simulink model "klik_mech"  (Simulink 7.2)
settings: Solver=ode45  StartTime=0.0  StopTime=10.0  MaxStep=0.05  RelTol=1e-3
InitFcn:
  | init_klik;
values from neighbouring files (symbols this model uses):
  L1 = 1.5    [init_klik.m]    (also in init_ctyrkloub.m = 3; init_withworth.m = 2)
  L2 = v/sin(uhel3)    [init_klik.m]    (also in init_ctyrkloub.m = 5; init_withworth.m = 5)
  L3 = L1/(sin(uhel1))    [init_klik.m]    (also in init_ctyrkloub.m = 0.5)
  omega = 5    [init_klik.m]    (also in init_ctyrkloub.m = 1; init_withworth.m = 0.5)
  uhel1 = (pi/180)*fi    (= 1.3962634016)    [init_klik.m]
undefined symbols (not defined in the file or in its folder): deg, kg, m, N, rad, s
libraries: mblibv1 x13, simulink x3

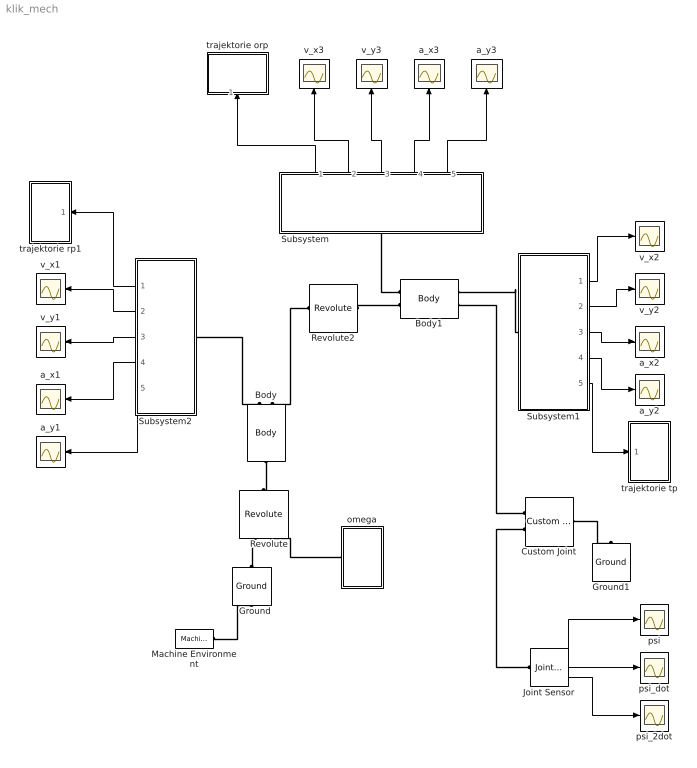
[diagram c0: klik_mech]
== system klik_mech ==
  Body : mblibv1/Bodies/Body  Orientation=up  DialogController=MECH.DynMechDlgSource  PhysicalDomain=mechanical  SubClassName=Unknown  LeftPortType=workingframe  RightPortType=workingframe  LConnTagsString=CS1  RConnTagsString=CS3|CS2  UpdateFromCAD=off  DialogClass=MechanicalBodyBlock  Mass=1  MassUnits=kg  InertiaUnits=kg*m^2  Inertia=eye(3)  Shape=Cylinder  ShapeDims=[1 1]  ShapeUnits=m  ShapeUse=false  Density=1  DensityUnits=kg/m^3  DensityUse=false  GraphicsMode=MACHINE_DEFAULT  BodyColorSelMode=MACHINE_DEFAULT  BodyColor=[1 0 0]  AttachedToCS=CG  CG=Left$CG$[L1/2 0 0]$CS1$CS1$m$[0 0 uhel1]$Euler X-Y-Z$rad$WORLD$false$none  WorkingFrames=Right$CS3$[0 0 0]$CS2$CS2$m$[0 0 uhel1]$Euler X-Y-Z$rad$WORLD$true$none#Left$CS1$[0 0 0]$Adjoining$Adjoining$m$[0 0 uhel1]$Euler X-Y-Z$rad$WORLD$true$none#Right$CS2$[L1 0 0]$CS1$CS1$m$[0 0 uhel1]$Euler X-Y-Z$rad$WORLD$true$none  CGPos=[L1/2 0 0]  CGRot=[0 0 uhel1]  CS0Pos=[]  CS0Rot=[]  CS1Pos=[0 0 0]  CS1Rot=[0 0 uhel1]  CS2Pos=[L1 0 0]  CS2Rot=[0 0 uhel1]  CS3Pos=[0 0 0]  CS3Rot=[0 0 uhel1]  CS4Pos=[]  CS4Rot=[]  CS5Pos=[]  CS5Rot=[]  CS6Pos=[]  CS6Rot=[]  CS7Pos=[]  CS7Rot=[]  CS8Pos=[]  CS8Rot=[]  CS9Pos=[]  CS9Rot=[]  CS10Pos=[]  CS10Rot=[]  CS11Pos=[]  CS11Rot=[]  CS12Pos=[]  CS12Rot=[]  CS13Pos=[]  CS13Rot=[]  CS14Pos=[]  CS14Rot=[]  CS15Pos=[]  CS15Rot=[]  CS16Pos=[]  CS16Rot=[]  CS17Pos=[]  CS17Rot=[]  CS18Pos=[]  CS18Rot=[]  CS19Pos=[]  CS19Rot=[]  CS20Pos=[]  CS20Rot=[]
  Body1 : mblibv1/Bodies/Body  DialogController=MECH.DynMechDlgSource  PhysicalDomain=mechanical  SubClassName=Unknown  LeftPortType=workingframe  RightPortType=workingframe  LConnTagsString=CG|CS1  RConnTagsString=CS3|CS2  UpdateFromCAD=off  DialogClass=MechanicalBodyBlock  Mass=1  MassUnits=kg  InertiaUnits=kg*m^2  Inertia=eye(3)  Shape=Cylinder  ShapeDims=[1 1]  ShapeUnits=m  ShapeUse=false  Density=1  DensityUnits=kg/m^3  DensityUse=false  GraphicsMode=MACHINE_DEFAULT  BodyColorSelMode=MACHINE_DEFAULT  BodyColor=[1 0 0]  AttachedToCS=CG  CG=Left$CG$[L2/2 0 0]$CS1$CS1$m$[0 0 0]$Euler X-Y-Z$rad$CS1$true$none  WorkingFrames=Right$CS3$[0 0 0]$CS2$CS2$m$[0 0 0]$Euler X-Y-Z$rad$CS1$true$none#Left$CS1$[0 0 0]$Adjoining$Adjoining$m$[0 0 3*pi/2]$Euler X-Y-Z$rad$Adjoining$true$none#Right$CS2$[L2 0 0]$CS1$CS1$m$[0 0 0]$Euler X-Y-Z$rad$CS1$true$none  CGPos=[L2/2 0 0]  CGRot=[0 0 0]  CS0Pos=[]  CS0Rot=[]  CS1Pos=[0 0 0]  CS1Rot=[0 0 3*pi/2]  CS2Pos=[L2 0 0]  CS2Rot=[0 0 0]  CS3Pos=[0 0 0]  CS3Rot=[0 0 0]  CS4Pos=[]  CS4Rot=[]  CS5Pos=[]  CS5Rot=[]  CS6Pos=[]  CS6Rot=[]  CS7Pos=[]  CS7Rot=[]  CS8Pos=[]  CS8Rot=[]  CS9Pos=[]  CS9Rot=[]  CS10Pos=[]  CS10Rot=[]  CS11Pos=[]  CS11Rot=[]  CS12Pos=[]  CS12Rot=[]  CS13Pos=[]  CS13Rot=[]  CS14Pos=[]  CS14Rot=[]  CS15Pos=[]  CS15Rot=[]  CS16Pos=[]  CS16Rot=[]  CS17Pos=[]  CS17Rot=[]  CS18Pos=[]  CS18Rot=[]  CS19Pos=[]  CS19Rot=[]  CS20Pos=[]  CS20Rot=[]
  Custom Joint : mblibv1/Joints/Custom Joint  DialogController=MECH.DynMechDlgSource  PhysicalDomain=mechanical  SubClassName=custom_joint  LeftPortType=blob  RightPortType=blob  LConnTagsString=__newl0|SA1  RConnTagsString=__newr0  UpdateFromCAD=off  NumSAPorts=1  CutJoint=off  MarkAsCut=off  Primitives=prismatic  PrimitiveProps=R1$World$[0 0 1]$Revolute#P1$World$[1 0 0]$Prismatic  DialogClass=JointBlock  R1Axis=[0 0 1]  R2Axis=[]  R3Axis=[]  P1Axis=[1 0 0]  P2Axis=[]  P3Axis=[]  SAxis=[]
  Ground : mblibv1/Bodies/Ground  Orientation=up  DialogController=MECH.DynMechDlgSource  SystemSampleTime=-1  UpdateFromCAD=off  LeftPortType=env  RightPortType=workingframe  PhysicalDomain=Mechanical  DialogClass=GroundBlock  CoordPosition=[0 0 0]  CoordPositionUnits=m  StateVectorMgrId=4  MachineId=[5 0]  ShowEnvPort=on
  Ground1 : mblibv1/Bodies/Ground  Orientation=up  DialogController=MECH.DynMechDlgSource  SystemSampleTime=-1  UpdateFromCAD=off  LeftPortType=env  RightPortType=workingframe  PhysicalDomain=Mechanical  DialogClass=GroundBlock  CoordPosition=[L3 0 0]  CoordPositionUnits=m  StateVectorMgrId=-1  MachineId=[0 0]  ShowEnvPort=off
  Joint Sensor : mblibv1/Sensors &  Actuators/Joint Sensor  DialogController=MECH.DynMechDlgSource  SystemSampleTime=-1  UpdateFromCAD=off  PhysicalDomain=Mechanical  PortType=blob  Muxed=off  Pose=off  Angle=on  AngleUnits=rad  ArcVelocity=on  ArcVelocityUnits=rad/s  ArcAcceleration=on  ArcAccelerationUnits=rad/s^2  CoordPosition=on  CoordPositionUnits=m  Velocity=off  VelocityUnits=m/s  Acceleration=off  AccelerationUnits=m/s^2  Quaternion=on  QuaternionDT=off  QuaternionDDT=off  QuaternionUnits=off  OutputVector=[1]  ActiveIO=on  Width=3  DialogClass=MechanicalSensorBlock  Primitive=R1  Force=off  ForceUnits=N  Torque=off  TorqueUnits=N*m  ReferenceFrame=Absolute (World)  ReactionSensedSide=Base  ReactionReferenceFrame=Absolute (World)  ReactionForce=off  ReactionForceUnits=N  ReactionMoment=off  ReactionMomentUnits=N*m
  Machine Environment : mblibv1/Bodies/Machine Environment  DialogController=MECH.DialogSource  SystemSampleTime=-1  PortType=env  PhysicalDomain=Mechanical  DialogTemplateClass=MECH.MachineEnvironment  SyncWhenCopied=off  Gravity=[0 -9.81 0]  GravityUnits=m/s^2  GravityAsSignal=off  Dimensionality=Auto-detect  AnalysisType=Kinematics  LinearAssemblyTolerance=1e-3  LinearAssemblyToleranceUnits=m  AngularAssemblyTolerance=1e-3  AngularAssemblyToleranceUnits=rad  ConstraintSolverType=Stabilizing  ConstraintRelTolerance=1e-4  ConstraintAbsTolerance=1e-4  UseRobustSingularityHandling=off  RedundancyAnalysisToleranceType=Automatically select tolerance  RedundancyAnalysisTolerance=1e-14  StatePerturbationType=Fixed  PerturbationSize=1e-5  VisualizeMachine=on  BodyVisualizationType=Use model default body geometries  BodyColorSelMode=Use model default  DefaultBodyColor=[1 0 0]
  Revolute : mblibv1/Joints/Revolute  Orientation=up  DialogController=MECH.DynMechDlgSource  PhysicalDomain=mechanical  SubClassName=Unknown  LeftPortType=blob  RightPortType=blob  LConnTagsString=__newl0|SA1  RConnTagsString=__newr0  UpdateFromCAD=off  NumSAPorts=1  CutJoint=off  MarkAsCut=off  Primitives=prismatic  PrimitiveProps=R1$World$[0 0 1]$revolute  DialogClass=JointBlock  R1Axis=[0 0 1]
  Revolute2 : mblibv1/Joints/Revolute  DialogController=MECH.DynMechDlgSource  PhysicalDomain=mechanical  SubClassName=Unknown  LeftPortType=blob  RightPortType=blob  LConnTagsString=__newl0  RConnTagsString=__newr0  UpdateFromCAD=off  NumSAPorts=0  CutJoint=off  MarkAsCut=off  Primitives=prismatic  PrimitiveProps=R1$WORLD$[0 0 1]$revolute  DialogClass=JointBlock  R1Axis=[0 0 1]
  Subsystem : Subsystem  Orientation=up
  Subsystem1 : Subsystem
  Subsystem2 : Subsystem  Orientation=left
  a_x1 : Scope
  a_x2 : Scope
  a_x3 : Scope
  a_y1 : Scope
  a_y2 : Scope
  a_y3 : Scope
  omega : Subsystem  Orientation=left
  psi : Scope
  psi_2dot : Scope
  psi_dot : Scope
  trajektorie orp : Subsystem  Orientation=up
  trajektorie rp1 : Subsystem  Orientation=left
  trajektorie tp : Subsystem
  v_x1 : Scope
  v_x2 : Scope
  v_x3 : Scope
  v_y1 : Scope
  v_y2 : Scope
  v_y3 : Scope
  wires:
  Joint Sensor/1 -> psi/1
  Subsystem1/1(Out1) -> v_x2/1
  Subsystem1/2(Out2) -> v_y2/1
  Subsystem1/3(Out3) -> a_x2/1
  Subsystem1/4(Out4) -> a_y2/1
  Subsystem1/5(Out5) -> trajektorie tp/1(In1)
  Subsystem/1(Out1) -> trajektorie orp/1(In1)
  Subsystem/2(Out2) -> v_x3/1
  Subsystem/3(Out3) -> v_y3/1
  Subsystem/4(Out4) -> a_x3/1
  Subsystem/5(Out5) -> a_y3/1
  Subsystem2/1(Out1) -> trajektorie rp1/1(In1)
  Subsystem2/2(Out2) -> v_x1/1
  Subsystem2/3(Out3) -> v_y1/1
  Subsystem2/4(Out4) -> a_x1/1
  Subsystem2/5(Out5) -> a_y1/1
  Joint Sensor/2 -> psi_dot/1
  Joint Sensor/3 -> psi_2dot/1
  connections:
  Subsystem2/LConn1 -- Body/RConn1
  Ground/RConn1 -- Revolute/LConn1
  omega/RConn1 -- Revolute/LConn2
  Subsystem/LConn1 -- Body1/LConn1
  Custom Joint/LConn1 -- Body1/RConn2
  Revolute2/LConn1 -- Body/RConn2
  Subsystem1/LConn1 -- Body1/RConn1
  Body/LConn1 -- Revolute/RConn1
  Revolute2/RConn1 -- Body1/LConn2
  Joint Sensor/LConn1 -- Custom Joint/LConn2
  Machine Environment/RConn1 -- Ground/LConn1
  Custom Joint/RConn1 -- Ground1/RConn1

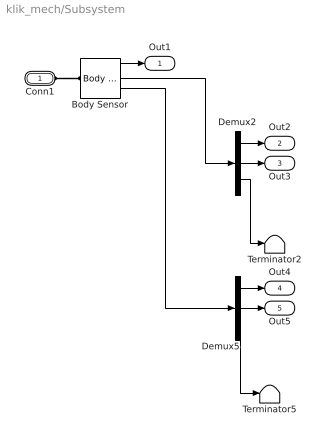
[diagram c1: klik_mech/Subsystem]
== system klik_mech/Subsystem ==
  Body Sensor : mblibv1/Sensors &  Actuators/Body Sensor  DialogController=MECH.DynMechDlgSource  SystemSampleTime=-1  UpdateFromCAD=off  PhysicalDomain=Mechanical  PortType=blob  Muxed=off  Pose=off  Angle=on  AngleUnits=deg  ArcVelocity=off  ArcVelocityUnits=deg/s  ArcAcceleration=off  ArcAccelerationUnits=deg/s^2  CoordPosition=on  CoordPositionUnits=m  Velocity=on  VelocityUnits=m/s  Acceleration=on  AccelerationUnits=m/s^2  Quaternion=on  QuaternionDT=off  QuaternionDDT=off  QuaternionUnits=off  OutputVector=[1]  ActiveIO=on  Width=9  DialogClass=MechanicalSensorBlock  ReferenceFrame=Absolute (World)
  Demux2 : Demux  Outputs=3
  Demux5 : Demux  Outputs=3
  Terminator2 : Terminator
  Terminator5 : Terminator
  Conn1 : PMIOPort  Port=1  Side=Left
  Out1 : Outport
  Out2 : Outport  Port=2
  Out3 : Outport  Port=3
  Out4 : Outport  Port=4
  Out5 : Outport  Port=5
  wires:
  Body Sensor/2 -> Demux2/1
  Demux2/3 -> Terminator2/1
  Demux5/3 -> Terminator5/1
  Body Sensor/3 -> Demux5/1
  Body Sensor/1 -> Out1/1
  Demux2/1 -> Out2/1
  Demux2/2 -> Out3/1
  Demux5/1 -> Out4/1
  Demux5/2 -> Out5/1
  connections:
  Conn1/RConn1 -- Body Sensor/LConn1

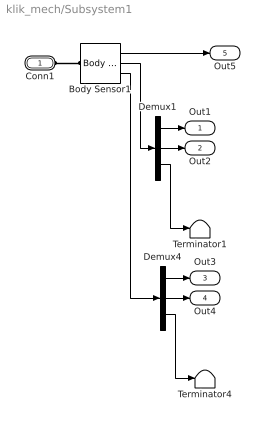
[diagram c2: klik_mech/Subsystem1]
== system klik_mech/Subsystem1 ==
  Body Sensor1 : mblibv1/Sensors &  Actuators/Body Sensor  DialogController=MECH.DynMechDlgSource  SystemSampleTime=-1  UpdateFromCAD=off  PhysicalDomain=Mechanical  PortType=blob  Muxed=off  Pose=off  Angle=on  AngleUnits=deg  ArcVelocity=off  ArcVelocityUnits=deg/s  ArcAcceleration=off  ArcAccelerationUnits=deg/s^2  CoordPosition=on  CoordPositionUnits=m  Velocity=on  VelocityUnits=m/s  Acceleration=on  AccelerationUnits=m/s^2  Quaternion=on  QuaternionDT=off  QuaternionDDT=off  QuaternionUnits=off  OutputVector=[1]  ActiveIO=on  Width=9  DialogClass=MechanicalSensorBlock  ReferenceFrame=Absolute (World)
  Demux1 : Demux  Outputs=3
  Demux4 : Demux  Outputs=3
  Terminator1 : Terminator
  Terminator4 : Terminator
  Conn1 : PMIOPort  Port=1  Side=Left
  Out1 : Outport
  Out2 : Outport  Port=2
  Out3 : Outport  Port=3
  Out4 : Outport  Port=4
  Out5 : Outport  Port=5
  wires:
  Body Sensor1/1 -> Out5/1
  Demux1/3 -> Terminator1/1
  Body Sensor1/2 -> Demux1/1
  Demux4/3 -> Terminator4/1
  Body Sensor1/3 -> Demux4/1
  Demux1/1 -> Out1/1
  Demux1/2 -> Out2/1
  Demux4/1 -> Out3/1
  Demux4/2 -> Out4/1
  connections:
  Conn1/RConn1 -- Body Sensor1/LConn1

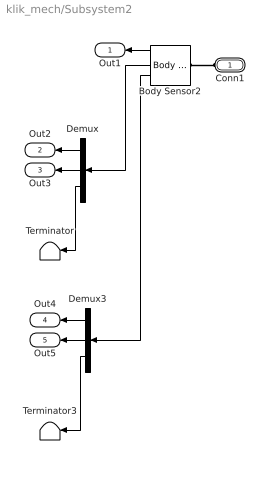
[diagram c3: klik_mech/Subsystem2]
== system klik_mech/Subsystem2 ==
  Body Sensor2 : mblibv1/Sensors &  Actuators/Body Sensor  Orientation=left  DialogController=MECH.DynMechDlgSource  SystemSampleTime=-1  UpdateFromCAD=off  PhysicalDomain=Mechanical  PortType=blob  Muxed=off  Pose=off  Angle=on  AngleUnits=deg  ArcVelocity=off  ArcVelocityUnits=deg/s  ArcAcceleration=off  ArcAccelerationUnits=deg/s^2  CoordPosition=on  CoordPositionUnits=m  Velocity=on  VelocityUnits=m/s  Acceleration=on  AccelerationUnits=m/s^2  Quaternion=on  QuaternionDT=off  QuaternionDDT=off  QuaternionUnits=off  OutputVector=[1]  ActiveIO=on  Width=9  DialogClass=MechanicalSensorBlock  ReferenceFrame=Absolute (World)
  Demux : Demux  Orientation=left  Outputs=3
  Demux3 : Demux  Orientation=left  Outputs=3
  Terminator : Terminator
  Terminator3 : Terminator
  Conn1 : PMIOPort  Orientation=left  Port=1  Side=Left
  Out1 : Outport  Orientation=left
  Out2 : Outport  Orientation=left  Port=2
  Out3 : Outport  Orientation=left  Port=3
  Out4 : Outport  Orientation=left  Port=4
  Out5 : Outport  Orientation=left  Port=5
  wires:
  Demux/3 -> Terminator/1
  Body Sensor2/2 -> Demux/1
  Demux3/3 -> Terminator3/1
  Body Sensor2/3 -> Demux3/1
  Body Sensor2/1 -> Out1/1
  Demux/1 -> Out2/1
  Demux/2 -> Out3/1
  Demux3/1 -> Out4/1
  Demux3/2 -> Out5/1
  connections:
  Conn1/RConn1 -- Body Sensor2/LConn1

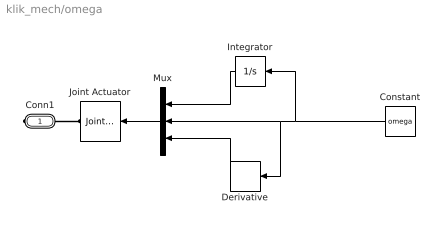
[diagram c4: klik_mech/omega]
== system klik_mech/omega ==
  Constant : Constant  Orientation=left  Value=omega  OutDataType=sfix(16)  OutScaling=2^0
  Derivative : Derivative  Orientation=left
  Integrator : Integrator  Orientation=left
  Joint Actuator : mblibv1/Sensors &  Actuators/Joint Actuator  Orientation=left  DialogController=MECH.DynMechDlgSource  SystemSampleTime=-1  UpdateFromCAD=off  PhysicalDomain=Mechanical  PortType=blob  ActuationStyle=Motion  AngleUnits=rad  ArcVelocityUnits=rad/s  ArcAccelerationUnits=rad/s^2  CoordPositionUnits=m  VelocityUnits=m/s  AccelerationUnits=m/s^2  ForceUnits=N  TorqueUnits=N*m  ActiveIO=on  Width=3  DialogClass=MechanicalActuatorBlock  Primitive=R1  ReferenceFrame=Absolute (World)
  Mux : Mux  Orientation=left  Inputs=3
  Conn1 : PMIOPort  Port=1  Side=Right
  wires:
  Constant/1 -> Derivative/1, Mux/2, Integrator/1
  Mux/1 -> Joint Actuator/1
  Integrator/1 -> Mux/1
  Derivative/1 -> Mux/3
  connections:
  Conn1/RConn1 -- Joint Actuator/RConn1

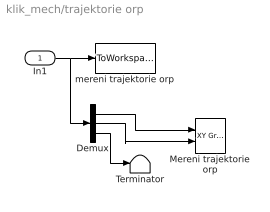
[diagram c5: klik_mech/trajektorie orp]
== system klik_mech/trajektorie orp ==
  In1 : Inport
  Demux : Demux  Outputs=3
  Mereni trajektorie orp : simulink/Sinks/XY Graph  SystemSampleTime=-1  xmin=2.5  xmax=6  ymin=-1  ymax=1  st=-1
  Terminator : Terminator
  mereni trajektorie orp : ToWorkspace  VariableName=orp  SampleTime=-1  SaveFormat=Array
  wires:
  In1/1 -> Demux/1, mereni trajektorie orp/1
  Demux/3 -> Terminator/1
  Demux/2 -> Mereni trajektorie orp/2
  Demux/1 -> Mereni trajektorie orp/1

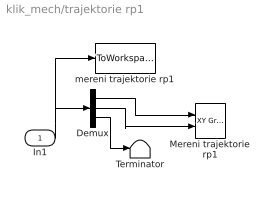
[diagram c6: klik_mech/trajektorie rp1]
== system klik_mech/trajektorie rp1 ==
  In1 : Inport
  Demux : Demux  Outputs=3
  Mereni trajektorie rp1 : simulink/Sinks/XY Graph  SystemSampleTime=-1  xmin=-3.3  xmax=3.3  ymin=-2.5  ymax=2.5  st=-1
  Terminator : Terminator
  mereni trajektorie rp1 : ToWorkspace  VariableName=rot  SampleTime=-1  SaveFormat=Array
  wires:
  Demux/1 -> Mereni trajektorie rp1/1
  Demux/2 -> Mereni trajektorie rp1/2
  Demux/3 -> Terminator/1
  In1/1 -> mereni trajektorie rp1/1, Demux/1

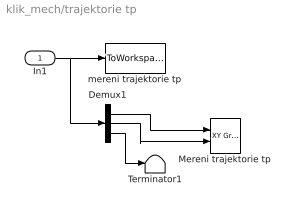
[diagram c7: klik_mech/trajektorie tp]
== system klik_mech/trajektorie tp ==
  In1 : Inport
  Demux1 : Demux  Outputs=3
  Mereni trajektorie tp : simulink/Sinks/XY Graph  SystemSampleTime=-1  xmin=6  xmax=11  ymin=-0.5  ymax=0.5  st=-1
  Terminator1 : Terminator
  mereni trajektorie tp : ToWorkspace  VariableName=trans  SampleTime=-1  SaveFormat=Array
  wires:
  In1/1 -> Demux1/1, mereni trajektorie tp/1
  Demux1/3 -> Terminator1/1
  Demux1/2 -> Mereni trajektorie tp/2
  Demux1/1 -> Mereni trajektorie tp/1
